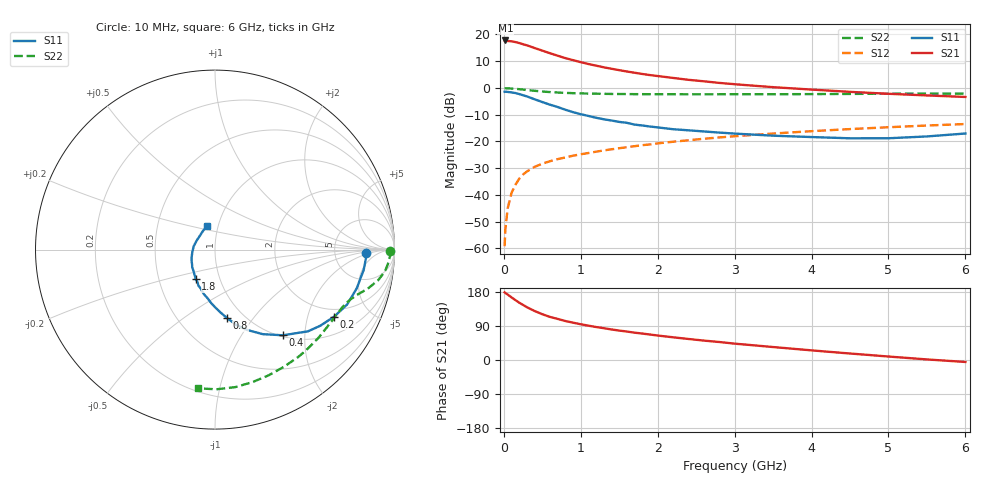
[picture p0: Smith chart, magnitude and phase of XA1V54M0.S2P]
! SIEMENS Discrete & RF Semiconductors
! BFY180
! Si NPN RF Bipolar Junction Transistor in MICRO-X
! VCE = 1.5 V  IC = 4 mA
! Common Emitter S-Parameters:  May  1997
# GHz  S  MA  R  50
!  f  S11  S21  S12  S22
! GHz  MAG  ANG  MAG  ANG  MAG  ANG  MAG  ANG
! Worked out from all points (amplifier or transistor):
!   36 points, 10 MHz to 6 GHz, reference 50 ohm
!   highest |S21| = 17.7 dB at 20 MHz (marker M1)
!   |S21| within 3 dB of that: start of sweep to 417.9 MHz
!   unconditionally stable (mu >= 1): 802.5 MHz to end of sweep
!   at 250 MHz: K = 0.39, MSG = 24.3 dB, |S12| = -32.4 dB
!   at 1.4 GHz: K = 1.29, MAG = 11.8 dB, |S12| = -23.0 dB
!   at 6 GHz: K = 1.33, MAG = 1.6 dB, |S12| = -13.5 dB
!   S11 on the Smith chart (normalised r, x): 10 MHz: 11, -2; 200 MHz: 1.67, -2.96; 400 MHz: 1.02, -1.55; 800 MHz: 0.84, -0.75; 1.8 GHz: 0.77, -0.26; 6 GHz: 0.89, +0.24
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0.01  0.8401 -1.4  7.509 178.5  0.0011 82.6  0.976 -0.3
0.02  0.8428 -3.0  7.648 176.8  0.0023 86.7  0.9792 -0.9
0.05  0.8361 -7.8  7.473 172.7  0.0056 82.9  0.975 -2.4
0.1  0.8186 -15.3  7.378 165.2  0.0109 81.8  0.967 -4.7
0.15  0.797 -22.6  7.145 158.1  0.0154 76.7  0.9565 -6.9
0.2  0.762 -29.3  6.842 151.3  0.02 73.1  0.9407 -8.8
0.25  0.7244 -35.8  6.496 145.3  0.024 70.2  0.9252 -10.6
0.3  0.6898 -41.3  6.206 139.3  0.0273 67.3  0.9067 -12.0
0.4  0.6092 -51.6  5.524 129.3  0.0333 62.7  0.8777 -14.4
0.5  0.5406 -60.6  4.938 120.8  0.0382 59.5  0.8508 -16.2
0.6  0.4826 -68.1  4.416 113.7  0.0425 57.7  0.8305 -17.7
0.8  0.3881 -79.9  3.573 102.8  0.0499 55.8  0.8021 -20.4
1  0.3207 -90.0  3.007 94.3  0.0573 54.2  0.785 -23.1
1.1  0.2977 -94.3  2.778 90.6  0.0604 53.8  0.7785 -24.4
1.4  0.2446 -106.8  2.264 80.6  0.0709 52.9  0.7666 -28.7
1.8  0.1973 -123.1  1.811 69.8  0.0847 51.4  0.7594 -34.5
2.2  0.1682 -135.7  1.527 59.9  0.0982 49.2  0.7575 -40.6
2.8  0.1455 -153.4  1.233 47.5  0.1181 45.7  0.7564 -49.5
3.5  0.1273 -173.6  1.026 34.2  0.1397 40.8  0.7576 -59.6
4.5  0.1138 153.6  0.839 17.1  0.1692 33.3  0.7673 -74.2
5.5  0.1233 123.3  0.719 1.5  0.1971 25.2  0.7783 -89.4
6  0.1399 107.5  0.673 -5.2  0.2102 21.0  0.7789 -97.1
